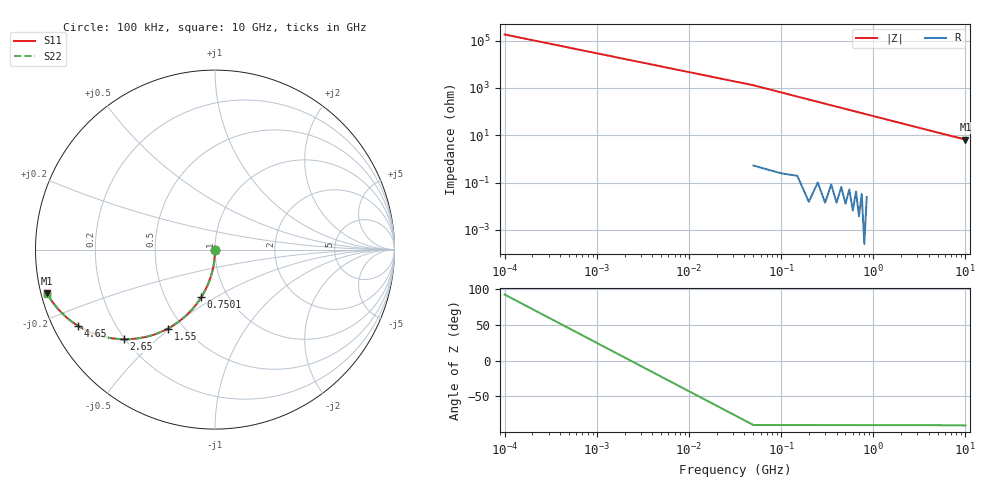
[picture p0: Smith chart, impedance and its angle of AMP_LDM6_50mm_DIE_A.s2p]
! Created Tue Aug  7 13:37:14 2007
# hz S ri R 50
! 2 Port Network Data from SP1.SP block
! freq  reS11  imS11  reS21  imS21  reS12  imS12  reS22  imS22
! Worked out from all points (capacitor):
!   201 points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, 100 kHz to 10 GHz, reference 50 ohm
!   read as one part in shunt: C = 2.44 pF near 50.1 MHz
!   lowest |Z| = 6.61 ohm at 10 GHz (marker M1)
!   S11 on the Smith chart (normalised r, x): 100 kHz: 1.00, +0.00; 750.1 MHz: 0.75, -0.43; 1.55 GHz: 0.41, -0.49; 2.65 GHz: 0.19, -0.40; 4.65 GHz: 0.07, -0.26; 10 GHz: 0.02, -0.13
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100000  2.09e-05 0.000111  1 0.000135  1 0.000135  2.36e-05 0.000165
5.01e7  -0.000341 -0.0186  0.9996 -0.0194  0.9996 -0.0194  -0.000339 -0.0193
1.001e8  -0.00146 -0.0385  0.9985 -0.0386  0.9985 -0.0386  -0.00147 -0.0385
1.501e8  -0.00329 -0.0569  0.9966 -0.0577  0.9966 -0.0577  -0.0033 -0.0575
2.001e8  -0.00585 -0.0765  0.9941 -0.0766  0.9941 -0.0766  -0.00585 -0.0764
3.001e8  -0.0131 -0.1138  0.9868 -0.1141  0.9868 -0.1141  -0.0131 -0.1137
4.001e8  -0.0231 -0.1503  0.9768 -0.1506  0.9768 -0.1506  -0.0231 -0.1502
5.001e8  -0.0356 -0.1853  0.9642 -0.1857  0.9642 -0.1857  -0.0356 -0.1852
7.501e8  -0.0767 -0.2654  0.923 -0.2667  0.923 -0.2667  -0.0767 -0.2659
9.001e8  -0.1069 -0.3088  0.8928 -0.3095  0.8928 -0.3095  -0.1069 -0.3087
1.1501e9  -0.1634 -0.3702  0.8362 -0.3704  0.8362 -0.3704  -0.1633 -0.3694
1.5501e9  -0.2618 -0.4399  0.7378 -0.4404  0.7378 -0.4404  -0.2616 -0.4392
1.7001e9  -0.299 -0.4574  0.7005 -0.4587  0.7005 -0.4587  -0.2988 -0.4574
2.0501e9  -0.3827 -0.4864  0.6167 -0.4871  0.6167 -0.4871  -0.3824 -0.4857
2.6501e9  -0.5088 -0.4993  0.4907 -0.5012  0.4907 -0.5012  -0.5083 -0.4997
3.3501e9  -0.6234 -0.4837  0.376 -0.4862  0.376 -0.4862  -0.6227 -0.4844
3.9501e9  -0.697 -0.4589  0.3024 -0.4614  0.3024 -0.4614  -0.6962 -0.4595
4.6501e9  -0.7612 -0.4256  0.2381 -0.4285  0.2381 -0.4285  -0.7604 -0.4264
5.0001e9  -0.7867 -0.4086  0.2126 -0.412  0.2126 -0.412  -0.7858 -0.4099
6.7001e9  -0.8687 -0.337  0.1304 -0.3409  0.1304 -0.3409  -0.8677 -0.3383
8.3501e9  -0.9114 -0.2832  0.0875 -0.2881  0.0875 -0.2881  -0.9104 -0.2852
1.00001e10  -0.9365 -0.2432  0.0621 -0.2484  0.0621 -0.2484  -0.9356 -0.2451
